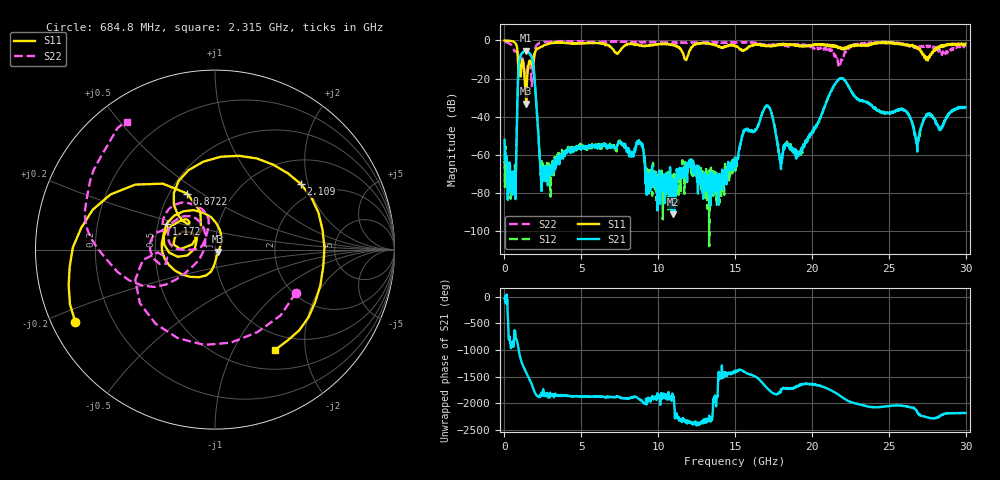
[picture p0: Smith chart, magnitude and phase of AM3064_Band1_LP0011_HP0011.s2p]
# Hz S DB R 50.0
!freq dBS11 angS11 dBS21 angS21 dBS12 angS12 dBS22 angS22
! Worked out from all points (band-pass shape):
!   1600 points, 10 MHz to 29.98 GHz, reference 50 ohm
!   highest |S21| = -5.35 dB at 1.397 GHz (marker M1); lowest = -91.2 dB at 10.98 GHz (marker M2)
!   |S21| within 3 dB of the highest: 1.032 GHz to 1.757 GHz (725.6 MHz wide, 52 % of centre)
!   lowest |S11| = -33.1 dB at 1.416 GHz (marker M3), VSWR 1.05, Z = 51.9 - j1.23 ohm
!   |S11| at or under -10 dB: 876.5 MHz to 1.914 GHz (1.038 GHz wide, 74.4 % of centre); 11.75 GHz to 11.84 GHz (89.31 MHz wide, 0.757 % of centre); 27.51051 GHz to 27.55348 GHz (42.97 MHz wide, 0.156 % of centre)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
!   |S22| runs from -24.0 to -0.3 dB; largest |S21 - S12| = 0.0057
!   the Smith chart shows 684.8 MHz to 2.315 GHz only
!   S11 on the Smith chart (normalised r, x): 684.8 MHz: 0.07, -0.24; 872.2 MHz: 0.61, +0.44; 1.172 GHz: 0.56, +0.18; 2.109 GHz: 1.58, +1.81; 2.315 GHz: 0.76, -1.48
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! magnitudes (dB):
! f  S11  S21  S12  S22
! 10 MHz  0.0  -52.1  -63.2  -0.3
! 684.8 MHz  -1.1  -75.7  -65.4  -5.8
! 872.2 MHz  -9.2  -22.9  -22.9  -9.9
! 1.172 GHz  -10.3  -6.6  -6.5  -9.5
! 1.397 GHz  -30.9  -5.4  -5.4  -21.9
! 1.416 GHz  -33.1  -5.4  -5.3  -20.9
! 1.809 GHz  -13.1  -9.6  -9.5  -20.5
! 2.109 GHz  -4.4  -38.0  -37.9  -2.3
! 2.315 GHz  -3.7  -63.9  -62.3  -1.3
! 5.015 GHz  -1.4  -55.8  -55.5  -0.6
! 8.763 GHz  -2.6  -54.1  -53.5  -1.1
! 9.326 GHz  -2.9  -69.5  -71.1  -0.9
! 10 GHz  -2.0  -75.9  -72.3  -0.9
! 10.98 GHz  -2.5  -91.2  -76.3  -1.0
! 15 GHz  -3.0  -66.3  -63.0  -1.2
! 17.05 GHz  -2.9  -34.4  -34.2  -2.8
! 17.97 GHz  -2.3  -61.4  -62.7  -2.1
! 19.99 GHz  -2.7  -48.2  -49.0  -3.4
! 21.87 GHz  -3.8  -19.9  -20.0  -11.3
! 25 GHz  -1.0  -38.1  -37.6  -1.1
! 26.83 GHz  -4.0  -55.4  -55.0  -3.5
! 29.98 GHz  -1.8  -35.0  -35.0  -3.2
